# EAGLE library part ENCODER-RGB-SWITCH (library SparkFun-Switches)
Illuminated Rotary Encoder w/ RGB LED and select switch Encoders rotate similarly to potentiometers, but they’re different from potentiometers in that an encoder has full rotation without limits. They output gray code so that you can tell how much and in which direction the encoder has been turned. This encoder includes an RGB LED and a push-down select switch. Part #: Top Up EC12PLRGBSDVBF-D SparkFun Products Rotary Encoder - Illuminated (RGB) (COM-10982)
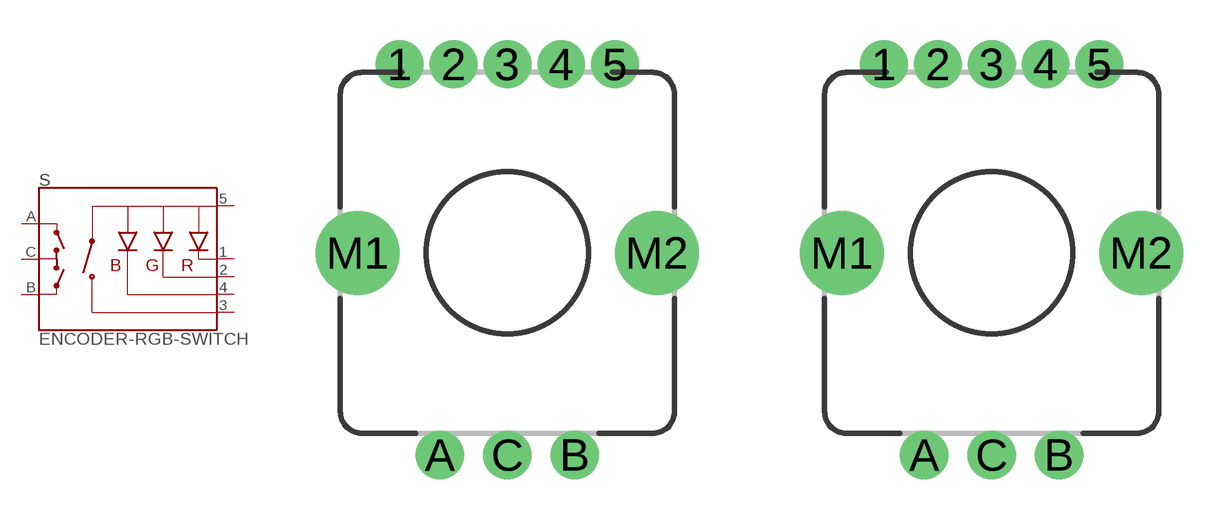
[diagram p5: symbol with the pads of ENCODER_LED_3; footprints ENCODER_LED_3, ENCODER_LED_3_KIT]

Designator prefix S

## ENCODER-RGB-SWITCH (PROD_ID: RES-10859; SF_SKU: COM-10982)  [ENCODER_LED_3]
1  -R  pas
2  -G  pas
3  SW  pas
4  -B  pas
5  +  pas
A  A
B  B
C  C

## ENCODER-RGB-SWITCHKIT (PROD_ID: RES-10859; SF_SKU: COM-10982)  [ENCODER_LED_3_KIT]
Pads as for ENCODER_LED_3

## Footprint ENCODER_LED_3 (pad centres in mm)
Illuminated Rotary Encoder w/ RGB LED and select switch Encoders rotate similarly to potentiometers, but they’re different from potentiometers in that an encoder has full rotation without limits.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
drill 1.1 pad 1.778: 1 -4,7; 2 -2,7; 3 0,7; 4 2,7; 5 4,7
drill 1.1 pad 1.8: A -2.5,-7.5; B 2.5,-7.5; C 0,-7.5
drill 2.1: M1 -5.55,0; M2 5.55,0

## Footprint ENCODER_LED_3_KIT (pad centres in mm)
Illuminated Rotary Encoder w/ RGB LED and select switch Encoders rotate similarly to potentiometers, but they’re different from potentiometers in that an encoder has full rotation without limits.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
drill 1.1 pad 1.778: 1 -4,7; 2 -2,7; 3 0,7; 4 2,7; 5 4,7
drill 1.1 pad 1.8: A -2.5,-7.5; B 2.5,-7.5; C 0,-7.5
drill 2.1: M1 -5.55,0; M2 5.55,0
